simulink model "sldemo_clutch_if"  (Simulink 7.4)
settings: Solver=ode23  SolverMode=SingleTasking  StartTime=0.0  StopTime=10  RelTol=1e-6  AbsTol=1e-7
PostLoadFcn:
  | % load the gui for plotting results
  | sldemo_clutchplot_if
StartFcn:
  | sldemo_clutchplot_if Start
StopFcn:
  | % See if logged data exists already
  | 
  | if exist ('sldemo_clutch_if_output')
  |    sldemo_clutchplot_if Stop
  | end
model workspace: external: M-Code (data not in the file)
undefined symbols (not defined in the file or in its folder): be, bv, Ie, Iv, muk, mus, R

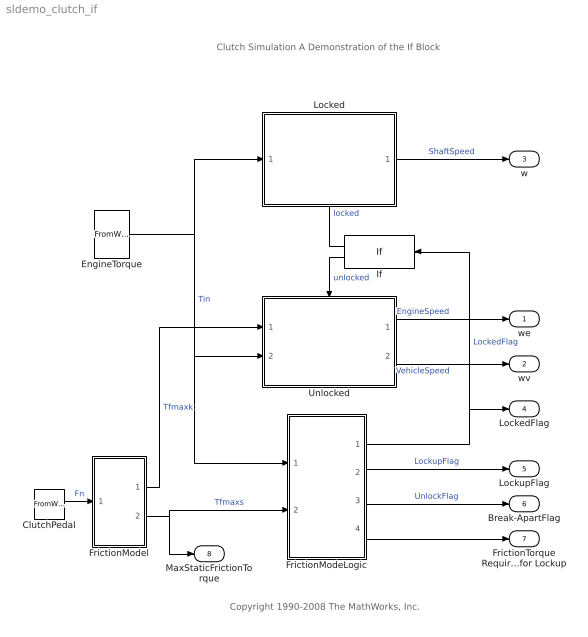
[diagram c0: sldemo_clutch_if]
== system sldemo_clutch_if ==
  note: Clutch Simulation A Demonstration of the If Block
  note: Copyright 1990-2008 The MathWorks, Inc.
  ClutchPedal : FromWorkspace  Description=|  VariableName=Fn  SampleTime=0
      | begin dimension                                                
      | output _ : [(length metre 1, mass kilogram 1, time second -2)];
      | end dimension
  EngineTorque : FromWorkspace  Description=|  VariableName=Tin  SampleTime=0
      | begin dimension                                                
      | output _ : [(length metre 2, mass kilogram 1, time second -2)];
      | end dimension
  FrictionModeLogic : Subsystem
  FrictionModel : Subsystem
  If : If
  Locked : Subsystem  TreatAsAtomicUnit=on
  Unlocked : Subsystem  TreatAsAtomicUnit=on
  we : Outport  Description=|  OutDataType=sfix(16)  OutScaling=2^0  InitialOutput=0
      | begin dimension              
      | input _ : [(time second -1)];
      | end dimension
  wv : Outport  Description=|  Port=2  OutDataType=sfix(16)  OutScaling=2^0  InitialOutput=0
      | begin dimension               
      | output _ : [(time second -1)];
      | end dimension
  w : Outport  Description=|  Port=3  OutDataType=sfix(16)  OutScaling=2^0  InitialOutput=0
      | begin dimension              
      | input _ : [(time second -1)];
      | end dimension
  LockedFlag : Outport  Description=|  Port=4  OutDataType=sfix(16)  OutScaling=2^0  InitialOutput=0
      | begin dimension             
      | input _ : [(dimensionless)];
      | end dimension
  LockupFlag : Outport  Description=|  Port=5  OutDataType=sfix(16)  OutScaling=2^0  InitialOutput=0
      | begin dimension             
      | input _ : [(dimensionless)];
      | end dimension
  Break-ApartFlag : Outport  Description=|  Port=6  OutDataType=sfix(16)  OutScaling=2^0  InitialOutput=0
      | begin dimension             
      | input _ : [(dimensionless)];
      | end dimension
  FrictionTorque Required for Lockup : Outport  Description=|  Port=7  OutDataType=sfix(16)  OutScaling=2^0  InitialOutput=0
      | begin dimension                                               
      | input _ : [(length metre 2, mass kilogram 1, time second -2)];
      | end dimension
  MaxStaticFrictionTorque : Outport  Description=|  Port=8  OutDataType=sfix(16)  OutScaling=2^0  InitialOutput=0
      | begin dimension                                               
      | input _ : [(length metre 2, mass kilogram 1, time second -2)];
      | end dimension
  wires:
  FrictionModeLogic/3(unlock) -> Break-ApartFlag/1  "UnlockFlag"
  FrictionModel/1(Tfmaxk) -> Unlocked/1(Tfmaxk)  "Tfmaxk"
  Unlocked/2(wv) -> wv/1  "VehicleSpeed"
  Unlocked/1(we) -> we/1  "EngineSpeed"
  FrictionModeLogic/1(locked) -> If/1, LockedFlag/1  "LockedFlag"
  FrictionModeLogic/2(lock) -> LockupFlag/1  "LockupFlag"
  FrictionModeLogic/4(Tf) -> FrictionTorque Required for Lockup/1
  Locked/1(w) -> w/1  "ShaftSpeed"
  FrictionModel/2(Tfmaxs) -> MaxStaticFrictionTorque/1, FrictionModeLogic/2(Tfmaxs)  "Tfmaxs"
  ClutchPedal/1 -> FrictionModel/1(Fn)  "Fn"
  EngineTorque/1 -> Locked/1(Tin), Unlocked/2(Tin), FrictionModeLogic/1(Tin)  "Tin"
  If/1 -> Locked/Action  "locked"
  If/2 -> Unlocked/Action  "unlocked"

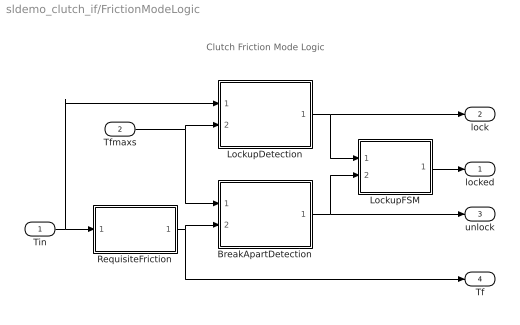
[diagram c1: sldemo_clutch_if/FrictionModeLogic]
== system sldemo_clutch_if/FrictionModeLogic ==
  note: Clutch Friction Mode Logic
  Tin : Inport  Description=|  OutDataType=sfix(16)  OutScaling=2^0
      | begin dimension                                                
      | output _ : [(length metre 2, mass kilogram 1, time second -2)];
      | end dimension
  Tfmaxs : Inport  Description=|  Port=2  OutDataType=sfix(16)  OutScaling=2^0
      | begin dimension                                                
      | output _ : [(length metre 2, mass kilogram 1, time second -2)];
      | end dimension
  BreakApartDetection : Subsystem
  LockupDetection : Subsystem
  LockupFSM : Subsystem
  RequisiteFriction : Subsystem
  locked : Outport  Description=|  OutDataType=sfix(16)  OutScaling=2^0  InitialOutput=0
      | begin dimension             
      | input _ : [(dimensionless)];
      | end dimension
  lock : Outport  Description=|  Port=2  OutDataType=sfix(16)  OutScaling=2^0  InitialOutput=0
      | begin dimension             
      | input _ : [(dimensionless)];
      | end dimension
  unlock : Outport  Description=|  Port=3  OutDataType=sfix(16)  OutScaling=2^0  InitialOutput=0
      | begin dimension             
      | input _ : [(dimensionless)];
      | end dimension
  Tf : Outport  Description=|  Port=4  OutDataType=sfix(16)  OutScaling=2^0  InitialOutput=0
      | begin dimension                                               
      | input _ : [(length metre 2, mass kilogram 1, time second -2)];
      | end dimension
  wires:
  Tin/1 -> LockupDetection/1(Tin), RequisiteFriction/1(Tin)
  Tfmaxs/1 -> LockupDetection/2(Tfmaxs), BreakApartDetection/1(Tfmaxs)
  RequisiteFriction/1(Tf) -> BreakApartDetection/2(Tf), Tf/1
  BreakApartDetection/1(unlock) -> LockupFSM/2(unlock), unlock/1
  LockupDetection/1(lock) -> LockupFSM/1(lock), lock/1
  LockupFSM/1(locked) -> locked/1

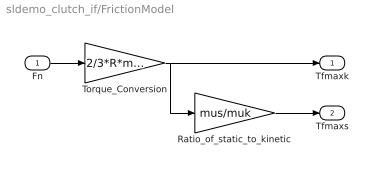
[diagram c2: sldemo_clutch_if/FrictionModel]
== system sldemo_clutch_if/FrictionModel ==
  Fn : Inport  Description=|  OutDataType=sfix(16)  OutScaling=2^0
      | begin dimension                                                
      | output _ : [(length metre 1, mass kilogram 1, time second -2)];
      | end dimension
  Ratio_of_static_to_kinetic : Gain  Description=|  Gain=mus/muk  ParameterDataType=sfix(16)  ParameterScaling=2^0  OutDataType=sfix(16)  OutScaling=2^0
      | begin dimension                
      | constant _ : [(dimensionless)];
      | end dimension
  Torque_Conversion : Gain  Description=|  Gain=2/3*R*muk  ParameterDataType=sfix(16)  ParameterScaling=2^0  OutDataType=sfix(16)  OutScaling=2^0
      | begin dimension                 
      | constant _ : [(length metre 1)];
      | end dimension
  Tfmaxk : Outport  Description=|  OutDataType=sfix(16)  OutScaling=2^0  InitialOutput=0
      | begin dimension                                               
      | input _ : [(length metre 2, mass kilogram 1, time second -2)];
      | end dimension
  Tfmaxs : Outport  Description=|  Port=2  OutDataType=sfix(16)  OutScaling=2^0  InitialOutput=0
      | begin dimension                                               
      | input _ : [(length metre 2, mass kilogram 1, time second -2)];
      | end dimension
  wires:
  Torque_Conversion/1 -> Tfmaxk/1, Ratio_of_static_to_kinetic/1
  Fn/1 -> Torque_Conversion/1
  Ratio_of_static_to_kinetic/1 -> Tfmaxs/1

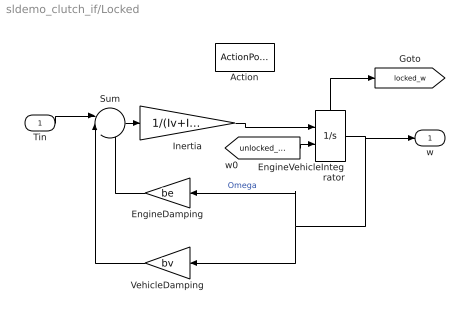
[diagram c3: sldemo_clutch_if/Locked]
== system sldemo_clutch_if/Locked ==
  Tin : Inport  Description=|  OutDataType=sfix(16)  OutScaling=2^0
      | begin dimension                                                
      | output _ : [(length metre 2, mass kilogram 1, time second -2)];
      | end dimension
  Action : ActionPort  InitializeStates=reset  ActionType=then
  EngineDamping : Gain  Description=|  Gain=be  ParameterDataType=sfix(16)  ParameterScaling=2^0  OutDataType=sfix(16)  OutScaling=2^0
      | begin dimension                                                  
      | constant _ : [(length metre 2, mass kilogram 1, time second -1)];
      | end dimension
  EngineVehicleIntegrator : Integrator  InitialConditionSource=external  ShowStatePort=on
  Inertia : Gain  Description=|  Gain=1/(Iv+Ie)  ParameterDataType=sfix(16)  ParameterScaling=2^0  OutDataType=sfix(16)  OutScaling=2^0
      | begin dimension                                    
      | constant _ : [(length metre -2, mass kilogram -1)];
      | end dimension
  Sum : Sum  Inputs=||+--  OutDataType=sfix(16)  OutScaling=2^0
  VehicleDamping : Gain  Description=|  Gain=bv  ParameterDataType=sfix(16)  ParameterScaling=2^0  OutDataType=sfix(16)  OutScaling=2^0
      | begin dimension                                                  
      | constant _ : [(length metre 2, mass kilogram 1, time second -1)];
      | end dimension
  w : Outport  Description=|  OutDataType=sfix(16)  OutScaling=2^0  InitialOutput=0
      | begin dimension              
      | input _ : [(time second -1)];
      | end dimension
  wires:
  [unlocked_we] -> EngineVehicleIntegrator/2
  EngineVehicleIntegrator/State -> [locked_w]
  Sum/1 -> Inertia/1
  Tin/1 -> Sum/1
  EngineVehicleIntegrator/1 -> w/1, EngineDamping/1, VehicleDamping/1  "Omega"
  EngineDamping/1 -> Sum/3
  Inertia/1 -> EngineVehicleIntegrator/1
  VehicleDamping/1 -> Sum/2

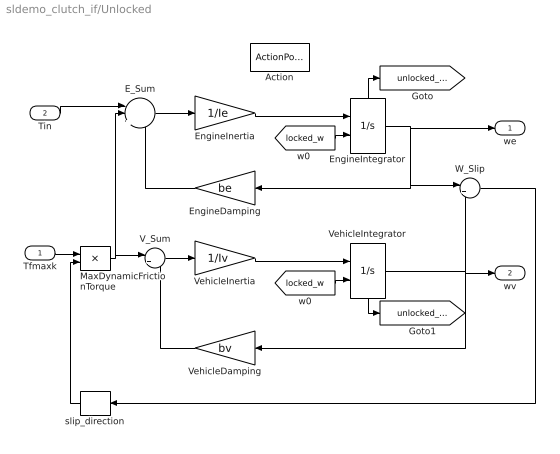
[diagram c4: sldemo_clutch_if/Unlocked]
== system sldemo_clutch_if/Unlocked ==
  Tfmaxk : Inport  Description=|  OutDataType=sfix(16)  OutScaling=2^0
      | begin dimension                                                
      | output _ : [(length metre 2, mass kilogram 1, time second -2)];
      | end dimension
  Tin : Inport  Description=|  Port=2  OutDataType=sfix(16)  OutScaling=2^0
      | begin dimension                                                
      | output _ : [(length metre 2, mass kilogram 1, time second -2)];
      | end dimension
  Action : ActionPort  InitializeStates=reset  ActionType=else
  E_Sum : Sum  Inputs=||+--  OutDataType=sfix(16)  OutScaling=2^0
  EngineDamping : Gain  Description=|  Gain=be  ParameterDataType=sfix(16)  ParameterScaling=2^0  OutDataType=sfix(16)  OutScaling=2^0
      | begin dimension                                                  
      | constant _ : [(length metre 2, mass kilogram 1, time second -1)];
      | end dimension
  EngineInertia : Gain  Description=|  Gain=1/Ie  ParameterDataType=sfix(16)  ParameterScaling=2^0  OutDataType=sfix(16)  OutScaling=2^0
      | begin dimension                                    
      | constant _ : [(length metre -2, mass kilogram -1)];
      | end dimension
  EngineIntegrator : Integrator  InitialConditionSource=external  ShowStatePort=on
  MaxDynamicFrictionTorque : Product  OutDataType=sfix(16)  OutScaling=2^0
  V_Sum : Sum  Inputs=|+-  OutDataType=sfix(16)  OutScaling=2^0
  VehicleDamping : Gain  Description=|  Gain=bv  ParameterDataType=sfix(16)  ParameterScaling=2^0  OutDataType=sfix(16)  OutScaling=2^0
      | begin dimension                                                
      | output _ : [(length metre 2, mass kilogram 1, time second -1)];
      | end dimension
  VehicleInertia : Gain  Description=|  Gain=1/Iv  ParameterDataType=sfix(16)  ParameterScaling=2^0  OutDataType=sfix(16)  OutScaling=2^0
      | begin dimension                                    
      | constant _ : [(length metre -2, mass kilogram -1)];
      | end dimension
  VehicleIntegrator : Integrator  InitialConditionSource=external  ShowStatePort=on
  W_Slip : Sum  Inputs=|+-  OutDataType=sfix(16)  OutScaling=2^0
  slip_direction : Signum
  we : Outport  Description=|  OutDataType=sfix(16)  OutScaling=2^0  InitialOutput=0
      | begin dimension              
      | input _ : [(time second -1)];
      | end dimension
  wv : Outport  Description=|  Port=2  OutDataType=sfix(16)  OutScaling=2^0  InitialOutput=0
      | begin dimension              
      | input _ : [(time second -1)];
      | end dimension
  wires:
  V_Sum/1 -> VehicleInertia/1
  VehicleDamping/1 -> V_Sum/2
  MaxDynamicFrictionTorque/1 -> V_Sum/1, E_Sum/2
  Tfmaxk/1 -> MaxDynamicFrictionTorque/1
  slip_direction/1 -> MaxDynamicFrictionTorque/2
  W_Slip/1 -> slip_direction/1
  EngineIntegrator/State -> [unlocked_we]
  EngineInertia/1 -> EngineIntegrator/1
  E_Sum/1 -> EngineInertia/1
  EngineDamping/1 -> E_Sum/3
  EngineIntegrator/1 -> we/1, EngineDamping/1, W_Slip/1
  [locked_w] -> EngineIntegrator/2
  Tin/1 -> E_Sum/1
  VehicleIntegrator/State -> [unlocked_wv]
  [locked_w] -> VehicleIntegrator/2
  VehicleInertia/1 -> VehicleIntegrator/1
  VehicleIntegrator/1 -> VehicleDamping/1, wv/1, W_Slip/2

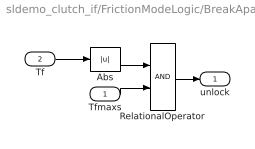
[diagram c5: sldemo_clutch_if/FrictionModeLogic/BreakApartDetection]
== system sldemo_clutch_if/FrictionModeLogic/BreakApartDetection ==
  Tfmaxs : Inport  Description=|  OutDataType=sfix(16)  OutScaling=2^0
      | begin dimension                                                
      | output _ : [(length metre 2, mass kilogram 1, time second -2)];
      | end dimension
  Tf : Inport  Description=|  Port=2  OutDataType=sfix(16)  OutScaling=2^0
      | begin dimension                                                
      | output _ : [(length metre 2, mass kilogram 1, time second -2)];
      | end dimension
  Abs : Abs
  RelationalOperator : RelationalOperator
  unlock : Outport  Description=|  OutDataType=sfix(16)  OutScaling=2^0  InitialOutput=0
      | begin dimension              
      | output _ : [(dimensionless)];
      | end dimension
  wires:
  Tf/1 -> Abs/1
  RelationalOperator/1 -> unlock/1
  Abs/1 -> RelationalOperator/1
  Tfmaxs/1 -> RelationalOperator/2

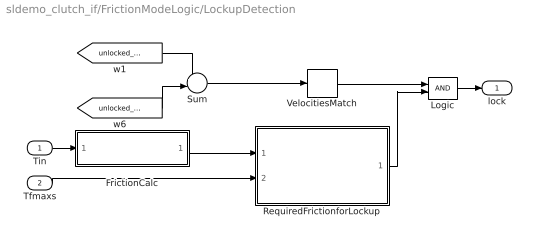
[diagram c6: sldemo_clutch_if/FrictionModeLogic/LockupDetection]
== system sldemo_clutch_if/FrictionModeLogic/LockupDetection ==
  Tin : Inport  Description=|  OutDataType=sfix(16)  OutScaling=2^0
      | begin dimension                                                
      | output _ : [(length metre 2, mass kilogram 1, time second -2)];
      | end dimension
  Tfmaxs : Inport  Description=|  Port=2  OutDataType=sfix(16)  OutScaling=2^0
      | begin dimension                                                
      | output _ : [(length metre 2, mass kilogram 1, time second -2)];
      | end dimension
  FrictionCalc : Subsystem
  Logic : Logic  IconShape=distinctive
  RequiredFrictionforLockup : Subsystem
  Sum : Sum  Inputs=+-  OutDataType=sfix(16)  OutScaling=2^0
  VelocitiesMatch : HitCross
  lock : Outport  Description=|  OutDataType=sfix(16)  OutScaling=2^0  InitialOutput=0
      | begin dimension             
      | input _ : [(dimensionless)];
      | end dimension
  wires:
  FrictionCalc/1(FrictionTorque) -> RequiredFrictionforLockup/1(FrictionTorque)
  Tfmaxs/1 -> RequiredFrictionforLockup/2(MaxFrictionTorque)
  VelocitiesMatch/1 -> Logic/1
  Logic/1 -> lock/1
  RequiredFrictionforLockup/1(okay) -> Logic/2
  [unlocked_we] -> Sum/1
  [unlocked_wv] -> Sum/2
  Sum/1 -> VelocitiesMatch/1
  Tin/1 -> FrictionCalc/1(Torque)

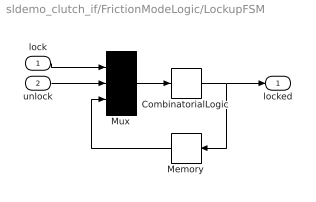
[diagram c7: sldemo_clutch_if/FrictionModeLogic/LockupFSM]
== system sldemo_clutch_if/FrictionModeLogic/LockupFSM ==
  lock : Inport  Description=|  OutDataType=sfix(16)  OutScaling=2^0
      | begin dimension              
      | output _ : [(dimensionless)];
      | end dimension
  unlock : Inport  Description=|  Port=2  OutDataType=sfix(16)  OutScaling=2^0
      | begin dimension              
      | output _ : [(dimensionless)];
      | end dimension
  CombinatorialLogic : CombinatorialLogic  TruthTable=[0;1;0;0;1;1;1;0]
  Memory : Memory
  Mux : Mux  Inputs=3
  locked : Outport  Description=|  OutDataType=sfix(16)  OutScaling=2^0  InitialOutput=0
      | begin dimension             
      | input _ : [(dimensionless)];
      | end dimension
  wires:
  Memory/1 -> Mux/3
  CombinatorialLogic/1 -> locked/1, Memory/1
  unlock/1 -> Mux/2
  lock/1 -> Mux/1
  Mux/1 -> CombinatorialLogic/1

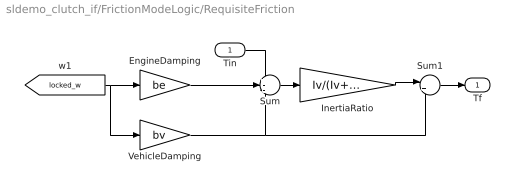
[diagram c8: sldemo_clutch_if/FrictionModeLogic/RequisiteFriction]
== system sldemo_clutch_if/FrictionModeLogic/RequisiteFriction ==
  Tin : Inport  Description=|  OutDataType=sfix(16)  OutScaling=2^0
      | begin dimension                                                
      | output _ : [(length metre 2, mass kilogram 1, time second -2)];
      | end dimension
  EngineDamping : Gain  Description=|  Gain=be  ParameterDataType=sfix(16)  ParameterScaling=2^0  OutDataType=sfix(16)  OutScaling=2^0
      | begin dimension                                                  
      | constant _ : [(length metre 2, mass kilogram 1, time second -1)];
      | end dimension
  InertiaRatio : Gain  Description=|  Gain=Iv/(Iv+Ie)  ParameterDataType=sfix(16)  ParameterScaling=2^0  OutDataType=sfix(16)  OutScaling=2^0
      | begin dimension                
      | constant _ : [(dimensionless)];
      | end dimension
  Sum : Sum  Inputs=+--  OutDataType=sfix(16)  OutScaling=2^0
  Sum1 : Sum  Inputs=|++  OutDataType=sfix(16)  OutScaling=2^0
  VehicleDamping : Gain  Description=|  Gain=bv  ParameterDataType=sfix(16)  ParameterScaling=2^0  OutDataType=sfix(16)  OutScaling=2^0
      | begin dimension                                                  
      | constant _ : [(length metre 2, mass kilogram 1, time second -1)];
      | end dimension
  Tf : Outport  Description=|  OutDataType=sfix(16)  OutScaling=2^0  InitialOutput=0
      | begin dimension                                               
      | input _ : [(length metre 2, mass kilogram 1, time second -2)];
      | end dimension
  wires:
  [locked_w] -> VehicleDamping/1, EngineDamping/1
  EngineDamping/1 -> Sum/2
  VehicleDamping/1 -> Sum/3, Sum1/2
  Sum/1 -> InertiaRatio/1
  Tin/1 -> Sum/1
  InertiaRatio/1 -> Sum1/1
  Sum1/1 -> Tf/1

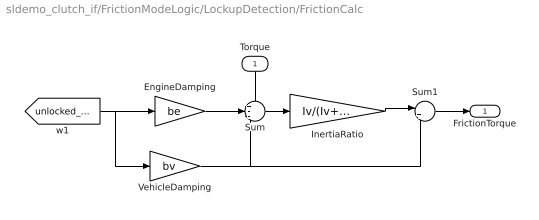
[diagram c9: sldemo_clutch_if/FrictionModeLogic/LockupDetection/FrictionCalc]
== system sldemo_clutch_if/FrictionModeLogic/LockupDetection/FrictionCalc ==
  Torque : Inport  Description=|  OutDataType=sfix(16)  OutScaling=2^0
      | begin dimension                                                
      | output _ : [(length metre 2, mass kilogram 1, time second -2)];
      | end dimension
  EngineDamping : Gain  Description=|  Gain=be  ParameterDataType=sfix(16)  ParameterScaling=2^0  OutDataType=sfix(16)  OutScaling=2^0
      | begin dimension                                                  
      | constant _ : [(length metre 2, mass kilogram 1, time second -1)];
      | end dimension
  InertiaRatio : Gain  Description=|  Gain=Iv/(Iv+Ie)  ParameterDataType=sfix(16)  ParameterScaling=2^0  OutDataType=sfix(16)  OutScaling=2^0
      | begin dimension                
      | constant _ : [(dimensionless)];
      | end dimension
  Sum : Sum  Inputs=+--  OutDataType=sfix(16)  OutScaling=2^0
  Sum1 : Sum  Inputs=|++  OutDataType=sfix(16)  OutScaling=2^0
  VehicleDamping : Gain  Description=|  Gain=bv  ParameterDataType=sfix(16)  ParameterScaling=2^0  OutDataType=sfix(16)  OutScaling=2^0
      | begin dimension                                                  
      | constant _ : [(length metre 2, mass kilogram 1, time second -1)];
      | end dimension
  FrictionTorque : Outport  Description=|  OutDataType=sfix(16)  OutScaling=2^0  InitialOutput=0
      | begin dimension                                               
      | input _ : [(length metre 2, mass kilogram 1, time second -2)];
      | end dimension
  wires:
  [unlocked_we] -> EngineDamping/1, VehicleDamping/1
  VehicleDamping/1 -> Sum1/2, Sum/3
  EngineDamping/1 -> Sum/2
  Sum/1 -> InertiaRatio/1
  Torque/1 -> Sum/1
  InertiaRatio/1 -> Sum1/1
  Sum1/1 -> FrictionTorque/1

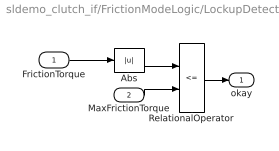
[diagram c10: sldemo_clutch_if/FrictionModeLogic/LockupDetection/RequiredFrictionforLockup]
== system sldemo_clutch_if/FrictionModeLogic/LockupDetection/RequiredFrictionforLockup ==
  FrictionTorque : Inport  Description=|  OutDataType=sfix(16)  OutScaling=2^0
      | begin dimension                                                
      | output _ : [(length metre 2, mass kilogram 1, time second -2)];
      | end dimension
  MaxFrictionTorque : Inport  Description=|  Port=2  OutDataType=sfix(16)  OutScaling=2^0
      | begin dimension                                                
      | output _ : [(length metre 2, mass kilogram 1, time second -2)];
      | end dimension
  Abs : Abs
  RelationalOperator : RelationalOperator  Operator=<=
  okay : Outport  Description=|  OutDataType=sfix(16)  OutScaling=2^0  InitialOutput=0
      | begin dimension             
      | input _ : [(dimensionless)];
      | end dimension
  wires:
  FrictionTorque/1 -> Abs/1
  RelationalOperator/1 -> okay/1
  Abs/1 -> RelationalOperator/1
  MaxFrictionTorque/1 -> RelationalOperator/2
